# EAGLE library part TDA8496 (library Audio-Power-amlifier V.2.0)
The UTC TDA8496 is a stereo 5+5W class AB power amplifier with mute and dc volume control, assembled in the HZIP-15A/B/D package. It is designed for high quality sound, LCD TV or LCD Monitor applications.
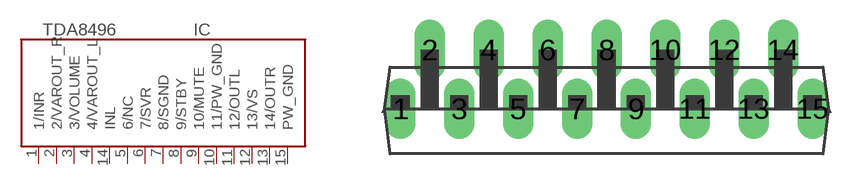
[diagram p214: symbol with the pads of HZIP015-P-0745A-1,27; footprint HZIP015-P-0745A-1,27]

Designator prefix IC

## TDA8496  [HZIP015-P-0745A-1,27]
1  1/INR  in
2  2/VAROUT_R  out
3  3/VOLUME  in
4  4/VAROUT_L  out
5  6/NC  nc
6  7/SVR
7  8/SGND  pwr
8  9/STBY  in
9  10/MUTE  in
10  11/PW_GND  pwr
11  12/OUTL  out
12  13/VS  pwr
13  14/OUTR  out
14  INL  in
15  PW_GND  pwr

## Footprint HZIP015-P-0745A-1,27 (pad centres in mm)
drill 0.8 long: 1 -8.89,-1.27; 2 -7.62,1.27; 3 -6.35,-1.27; 4 -5.08,1.27; 5 -3.81,-1.27; 6 -2.54,1.27; 7 -1.27,-1.27; 8 0,1.27; 9 1.27,-1.27; 10 2.54,1.27; 11 3.81,-1.27; 12 5.08,1.27; 13 6.35,-1.27; 14 7.62,1.27; 15 8.89,-1.27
